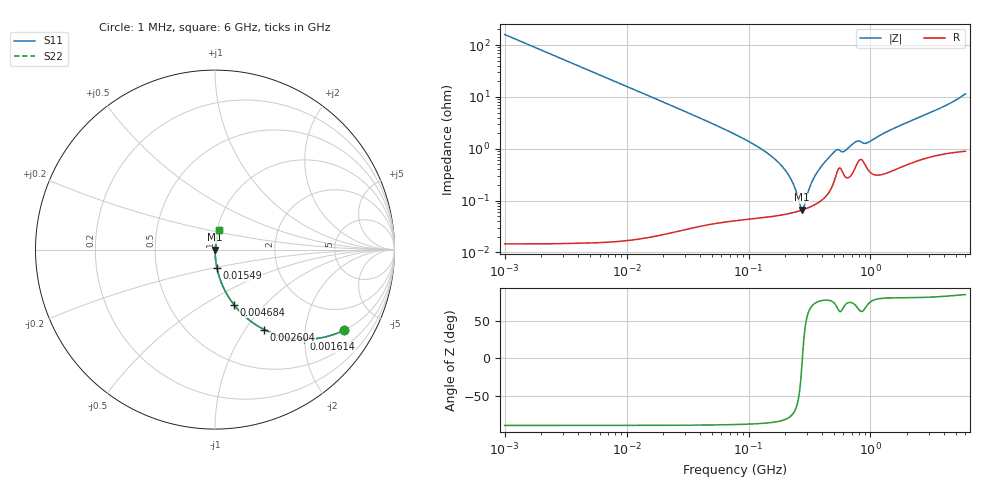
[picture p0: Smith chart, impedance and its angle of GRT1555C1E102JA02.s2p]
!Murata Part Number: GRT1555C1E102JA02
!These Parameters are Measured in Series Mode Connection
!Data Generated on Jun 19, 2026
!  o--ll--o
!Port1  Port2
!  o------o
!Operation Temp=25[degC], DC Bias Voltage=0[V]
!Freq. Start=1000[kHz] Stop=6[GHz] 401[Steps]
# Hz S RI R 50
!Freq.(Hz) S11(Real) S11(Imag) S21(Real) S21(Imag) S12(Real) S12(Imag) S22(Real) S22(Imag)
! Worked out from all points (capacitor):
!   401 points, 1 MHz to 6 GHz, reference 50 ohm
!   read as one part in series: C = 993 pF near 1.044 MHz
!   lowest |Z| = 66.7 mohm at 273.5 MHz (marker M1)
!   series resonance near 276.4 MHz, so ESL is about 330 pH
!   S11 on the Smith chart (normalised r, x): 1 MHz: 1.00, -3.21; 1.614 MHz: 1.00, -1.99; 2.604 MHz: 1.00, -1.23; 4.684 MHz: 1.00, -0.68; 15.49 MHz: 1.00, -0.21; 6 GHz: 1.02, +0.23
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1000000  0.7197 -0.4491  0.2803 0.4491  0.2803 0.4491  0.7197 -0.4491
1613609  0.4966 -0.4999  0.5034 0.4999  0.5034 0.4999  0.4966 -0.4999
2603734  0.2748 -0.4463  0.7252 0.4463  0.7252 0.4463  0.2748 -0.4463
4293785  0.1223 -0.3274  0.8777 0.3274  0.8777 0.3274  0.1223 -0.3274
4684054  0.1048 -0.3061  0.8952 0.3061  0.8952 0.3061  0.1048 -0.3061
1.549236e7  0.0107 -0.1019  0.9893 0.1019  0.9893 0.1019  0.0107 -0.1019
1.843659e7  0.00762 -0.0858  0.9924 0.0858  0.9924 0.0858  0.00762 -0.0858
7.745967e7  0.000768 -0.019  0.9992 0.019  0.9992 0.019  0.000768 -0.019
1.305463e8  0.000558 -0.00951  0.9994 0.00951  0.9994 0.00951  0.000558 -0.00951
1.848803e8  0.000548 -0.0048  0.9995 0.0048  0.9995 0.0048  0.000548 -0.0048
2.248532e8  0.000582 -0.00242  0.9994 0.00242  0.9994 0.00242  0.000582 -0.00242
2.734687e8  0.000655 -0.000124  0.9993 0.000124  0.9993 0.000124  0.000655 -0.000124
2.856264e8  0.000678 0.000388  0.9993 -0.000388  0.9993 -0.000388  0.000678 0.000388
3.325952e8  0.00079 0.00222  0.9992 -0.00222  0.9992 -0.00222  0.00079 0.00222
3.958029e8  0.00102 0.00448  0.999 -0.00448  0.999 -0.00448  0.00102 0.00448
5.138348e8  0.0028 0.00863  0.9972 -0.00863  0.9972 -0.00863  0.0028 0.00863
6.11486e8  0.00307 0.00843  0.9969 -0.00843  0.9969 -0.00843  0.00307 0.00843
7.767579e8  0.00526 0.0129  0.9947 -0.0129  0.9947 -0.0129  0.00526 0.0129
9.447004e8  0.00422 0.0123  0.9958 -0.0123  0.9958 -0.0123  0.00422 0.0123
1.428092e9  0.00403 0.0221  0.996 -0.0221  0.996 -0.0221  0.00403 0.0221
3.800129e9  0.0113 0.0604  0.9887 -0.0604  0.9887 -0.0604  0.0113 0.0604
6e9  0.0215 0.111  0.9785 -0.111  0.9785 -0.111  0.0215 0.111
